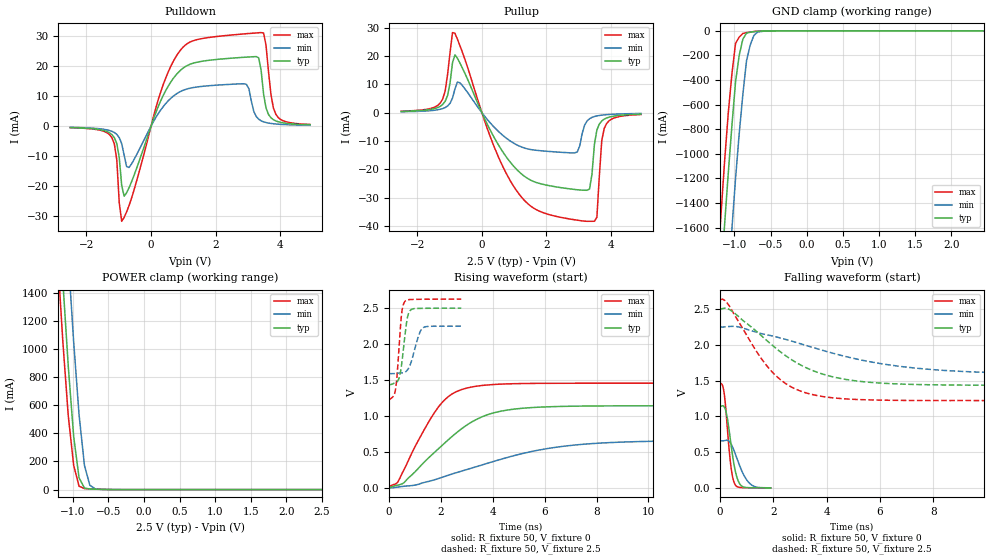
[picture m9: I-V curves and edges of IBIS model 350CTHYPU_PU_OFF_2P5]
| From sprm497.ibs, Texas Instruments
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|   Model Cell 350CTHYPU_PU_OFF_2P5
|BC3350CTHYPU_PU_OFF_2P5
[Model]   350CTHYPU_PU_OFF_2P5
Model_type   I/O
Polarity   Non-Inverting
Enable   Active-Low
Vinl =  0.7V
Vinh =  1.7V
Cref =  15.0000pF
Rref =  100.0000M
Vref =  0V
Vmeas =  1.25
C_comp   1.471008p   1.454665p   1.48896p
[Model Spec]
Vinl   0.7V   0.7V   0.7V
Vinh   1.7V   1.7V   1.7V
[Temperature Range]   25   125   -40
[Voltage Range]   2.5   2.25   2.625
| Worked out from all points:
|   slope of the pulldown table from 0 to 0.375 V, typ, clamps not added: 36.8 ohm
|   slope of the pullup table from 0 to 0.375 V, typ, clamps not added: 43.3 ohm
|   GND clamp passes 1 mA (typ) near -0.58 V on its own axis
|   POWER clamp passes 1 mA (typ) near -0.52 V on its own axis
|   rising waveform, R_fixture 50, V_fixture 0: 20-80 % time 2.16ns typ, 3.85ns min, 1.35ns max; typ from 0.002 V to 1.14 V
|   rising waveform, R_fixture 50, V_fixture 2.5: 20-80 % time 214ps typ, 317ps min, 169ps max; typ from 1.43 V to 2.5 V
|   falling waveform, R_fixture 50, V_fixture 0: 20-80 % time 277ps typ, 443ps min, 210ps max; typ from 1.14 V to 0.001 V
|   falling waveform, R_fixture 50, V_fixture 2.5: 20-80 % time 2.38ns typ, 4.27ns min, 1.64ns max; typ from 2.5 V to 1.43 V
[POWER_clamp]
|   voltage   I(typ)   I(min)   I(max)
-2.5V     14.49A     15.27A     14.05A
-1.187V   1.915A     2.738A     1.465A
-1.162V   1.698A     2.516A     1.258A
-1.136V   1.481A     2.293A     1.051A
-1.111V   1.28A      2.079A     875.8mA
-1.035V   711.3mA    1.451A     408.3mA
-984.8mV  377.9mA    1.051A     173mA
-909.1mV  83.51mA    532.5mA    24.23mA
-833.3mV  11.44mA    171.8mA    7.269mA
-757.6mV  4.356mA    30.73mA    5.048mA
-681.8mV  2.869mA    5.089mA    3.482mA
2.5V      127.5pA    9.115nA    3.788pA
[Pulldown]
|   voltage   I(typ)   I(min)   I(max)
-2.5V     -481.1uA   -397.3uA   -508.7uA
-1.212V   -2.823mA   -1.735mA   -3.853mA
-1.061V   -5.827mA   -2.764mA   -11.27mA
-909.1mV  -19.76mA   -5.838mA   -31.7mA
-681.8mV  -20.51mA   -13.77mA   -26.47mA
378.8mV   10.27mA    6.528mA    13.88mA
1.212V    20.63mA    12.64mA    28.03mA
2.955V    22.98mA    13.91mA    30.79mA
3.258V    23.15mA    3.189mA    31.03mA
3.485V    10.6mA     1.427mA    31.01mA
3.864V    1.733mA    710uA      3.928mA
4.924V    445.6uA    287.2uA    553.5uA
[Pullup]
|   voltage   I(typ)   I(min)   I(max)
-2.5V     459.9uA    322.6uA    529.5uA
-1.288V   2.256mA    1.218mA    3.421mA
-1.061V   6.152mA    2.378mA    13.64mA
-909.1mV  17.71mA    5.195mA    28.32mA
-833.3mV  20.44mA    8.44mA     28.06mA
1.061V    -19.86mA   -11.24mA   -27.34mA
2.879V    -27.14mA   -14.19mA   -37.86mA
3.258V    -27.41mA   -2.905mA   -38.38mA
3.561V    -6.117mA   -1.138mA   -36.93mA
3.712V    -2.921mA   -859.9uA   -9.775mA
3.864V    -1.868mA   -689uA     -3.792mA
4.924V    -509.7uA   -284.1uA   -641.8uA
[GND_clamp]
|   voltage   I(typ)   I(min)   I(max)
-2.5V     -14.63A    -15.47A    -14.16A
-1.237V   -2.471A    -3.372A    -1.946A
-1.187V   -2.02A     -2.917A    -1.498A
-1.136V   -1.576A    -2.468A    -1.061A
-1.035V   -772.8mA   -1.611A    -351.9mA
-984.8mV  -415.6mA   -1.202A    -102.1mA
-934.3mV  -199.9mA   -837.3mA   -50.88mA
-883.8mV  -67.48mA   -518.4mA   -21.68mA
-833.3mV  -18.31mA   -244.8mA   -14.52mA
-782.8mV  -11.52mA   -117mA     -10.03mA
-681.8mV  -3.837mA   -10.59mA   -3.106mA
2.449V    -729.8pA   2.28uA     -25.62pA
[Ramp]
| variable   typ   min   max
dV/dt_f  0.6473111/2.401895n   0.40306/4.35333n   0.8514772/1.649968n
dV/dt_r   0.684955/2.159123n   0.3951671/3.874543n   0.8729796/1.363677n
R_load = 50
[Rising Waveform]
R_fixture = 50
V_fixture = 0
V_fixture_min = 0
V_fixture_max = 0
|   time   V(typ)   V(min)   V(max)
0s        2.16mV     -451uV     16.15mV
330ps     38.01mV    10.33mV    76.35mV
576ps     71.5mV     22.13mV    254.4mV
1.155ns   282.5mV    51.17mV    678.9mV
1.899ns   542.6mV    128.8mV    1.123V
2.337ns   685.7mV    181.8mV    1.283V
2.925ns   855.3mV    246.9mV    1.38V
4.335ns   1.067V     399.5mV    1.442V
7.194ns   1.135V     596.5mV    1.454V
14.3ns    1.141V     655.9mV    1.455V
[Rising Waveform]
R_fixture = 50
V_fixture = 2.5
V_fixture_min = 2.25
V_fixture_max = 2.625
|   time   V(typ)   V(min)   V(max)
0s        1.434V     1.588V     1.225V
246ps     1.462V     1.59V      1.37V
303ps     1.474V     1.593V     1.553V
381ps     1.526V     1.596V     1.948V
477ps     1.705V     1.598V     2.408V
600ps     2.089V     1.607V     2.589V
687ps     2.333V     1.631V     2.612V
780ps     2.451V     1.685V     2.617V
1.272ns   2.496V     2.217V     2.622V
2.781ns   2.498V     2.248V     2.624V
[Falling Waveform]
R_fixture = 50
V_fixture = 0
V_fixture_min = 0
V_fixture_max = 0
|   time   V(typ)   V(min)   V(max)
0s        1.141V     658.3mV    1.456V
120ps     1.146V     658.5mV    1.401V
222ps     1.072V     666mV      1.087V
393ps     665.7mV    628.4mV    353.3mV
468ps     461.6mV    574.8mV    163.1mV
552ps     275.6mV    497.4mV    56.36mV
654ps     126.8mV    394mV      15.81mV
768ps     42.89mV    282mV      5.738mV
1.119ns   3.225mV    61.64mV    1.755mV
1.899ns   1.217mV    2.268mV    890.3uV
[Falling Waveform]
R_fixture = 50
V_fixture = 2.5
V_fixture_min = 2.25
V_fixture_max = 2.625
|   time   V(typ)   V(min)   V(max)
0s        2.499V     2.25V      2.632V
192ps     2.513V     2.251V     2.617V
384ps     2.487V     2.258V     2.526V
1.437ns   2.166V     2.169V     1.869V
2.01ns    1.979V     2.12V      1.6V
2.691ns   1.791V     2.052V     1.408V
3.564ns   1.628V     1.954V     1.297V
5.295ns   1.488V     1.788V     1.234V
8.154ns   1.441V     1.649V     1.221V
17.4ns    1.434V     1.59V      1.221V
